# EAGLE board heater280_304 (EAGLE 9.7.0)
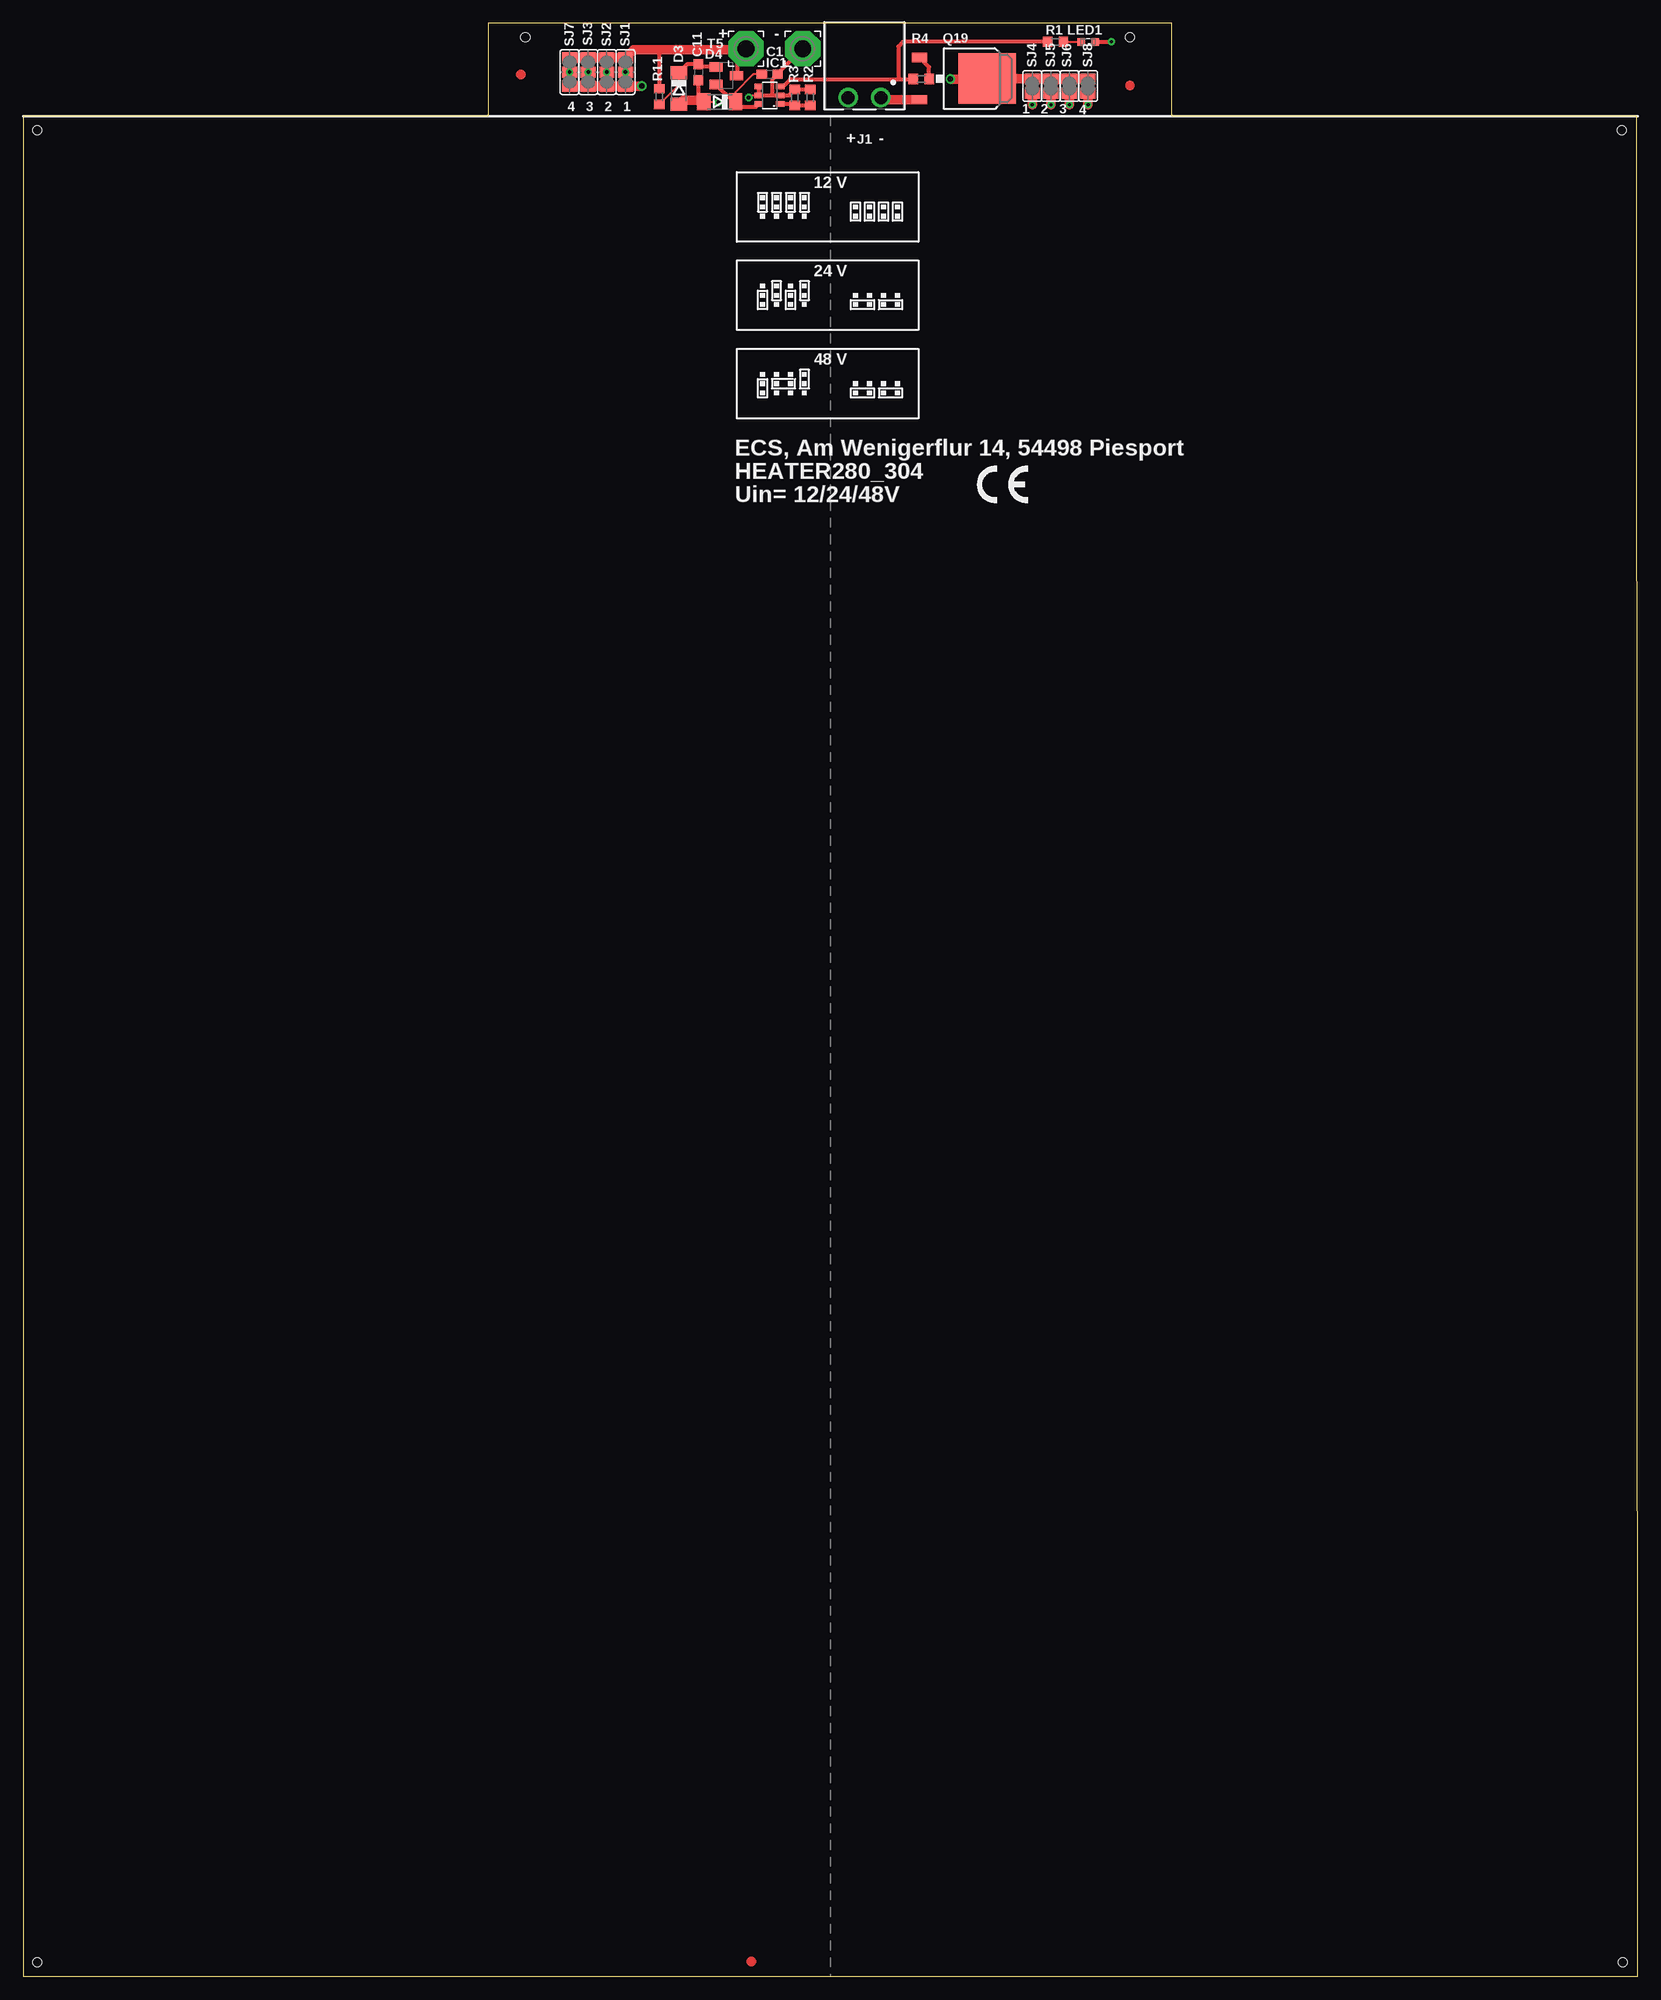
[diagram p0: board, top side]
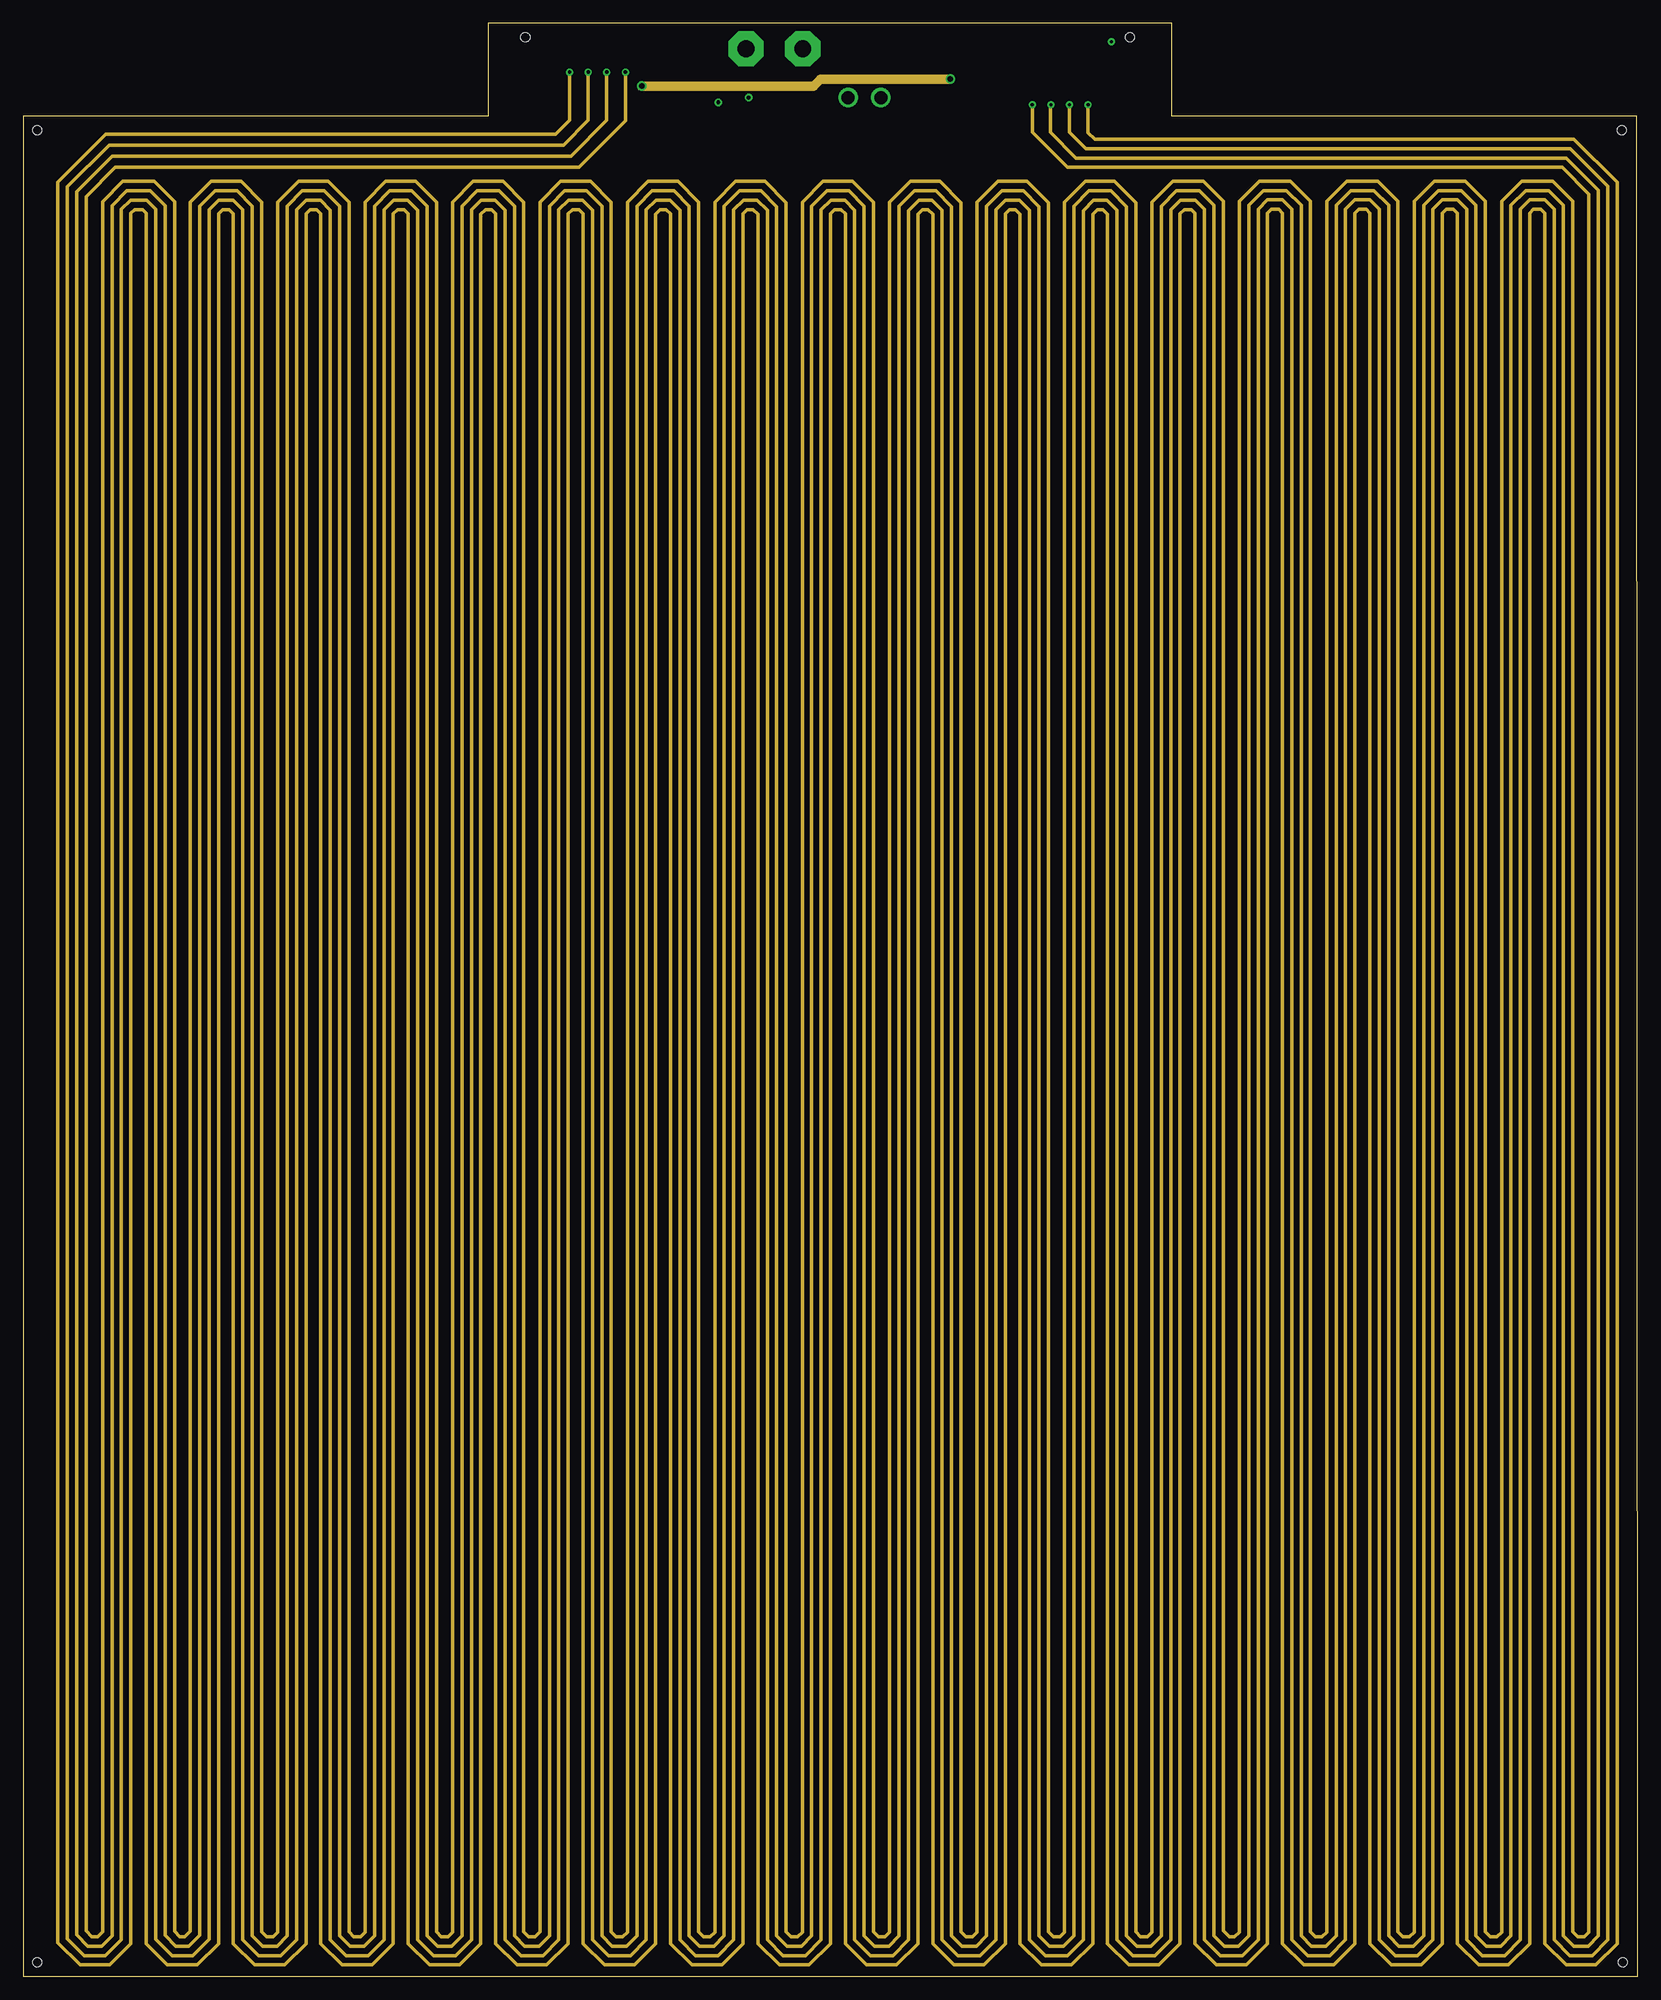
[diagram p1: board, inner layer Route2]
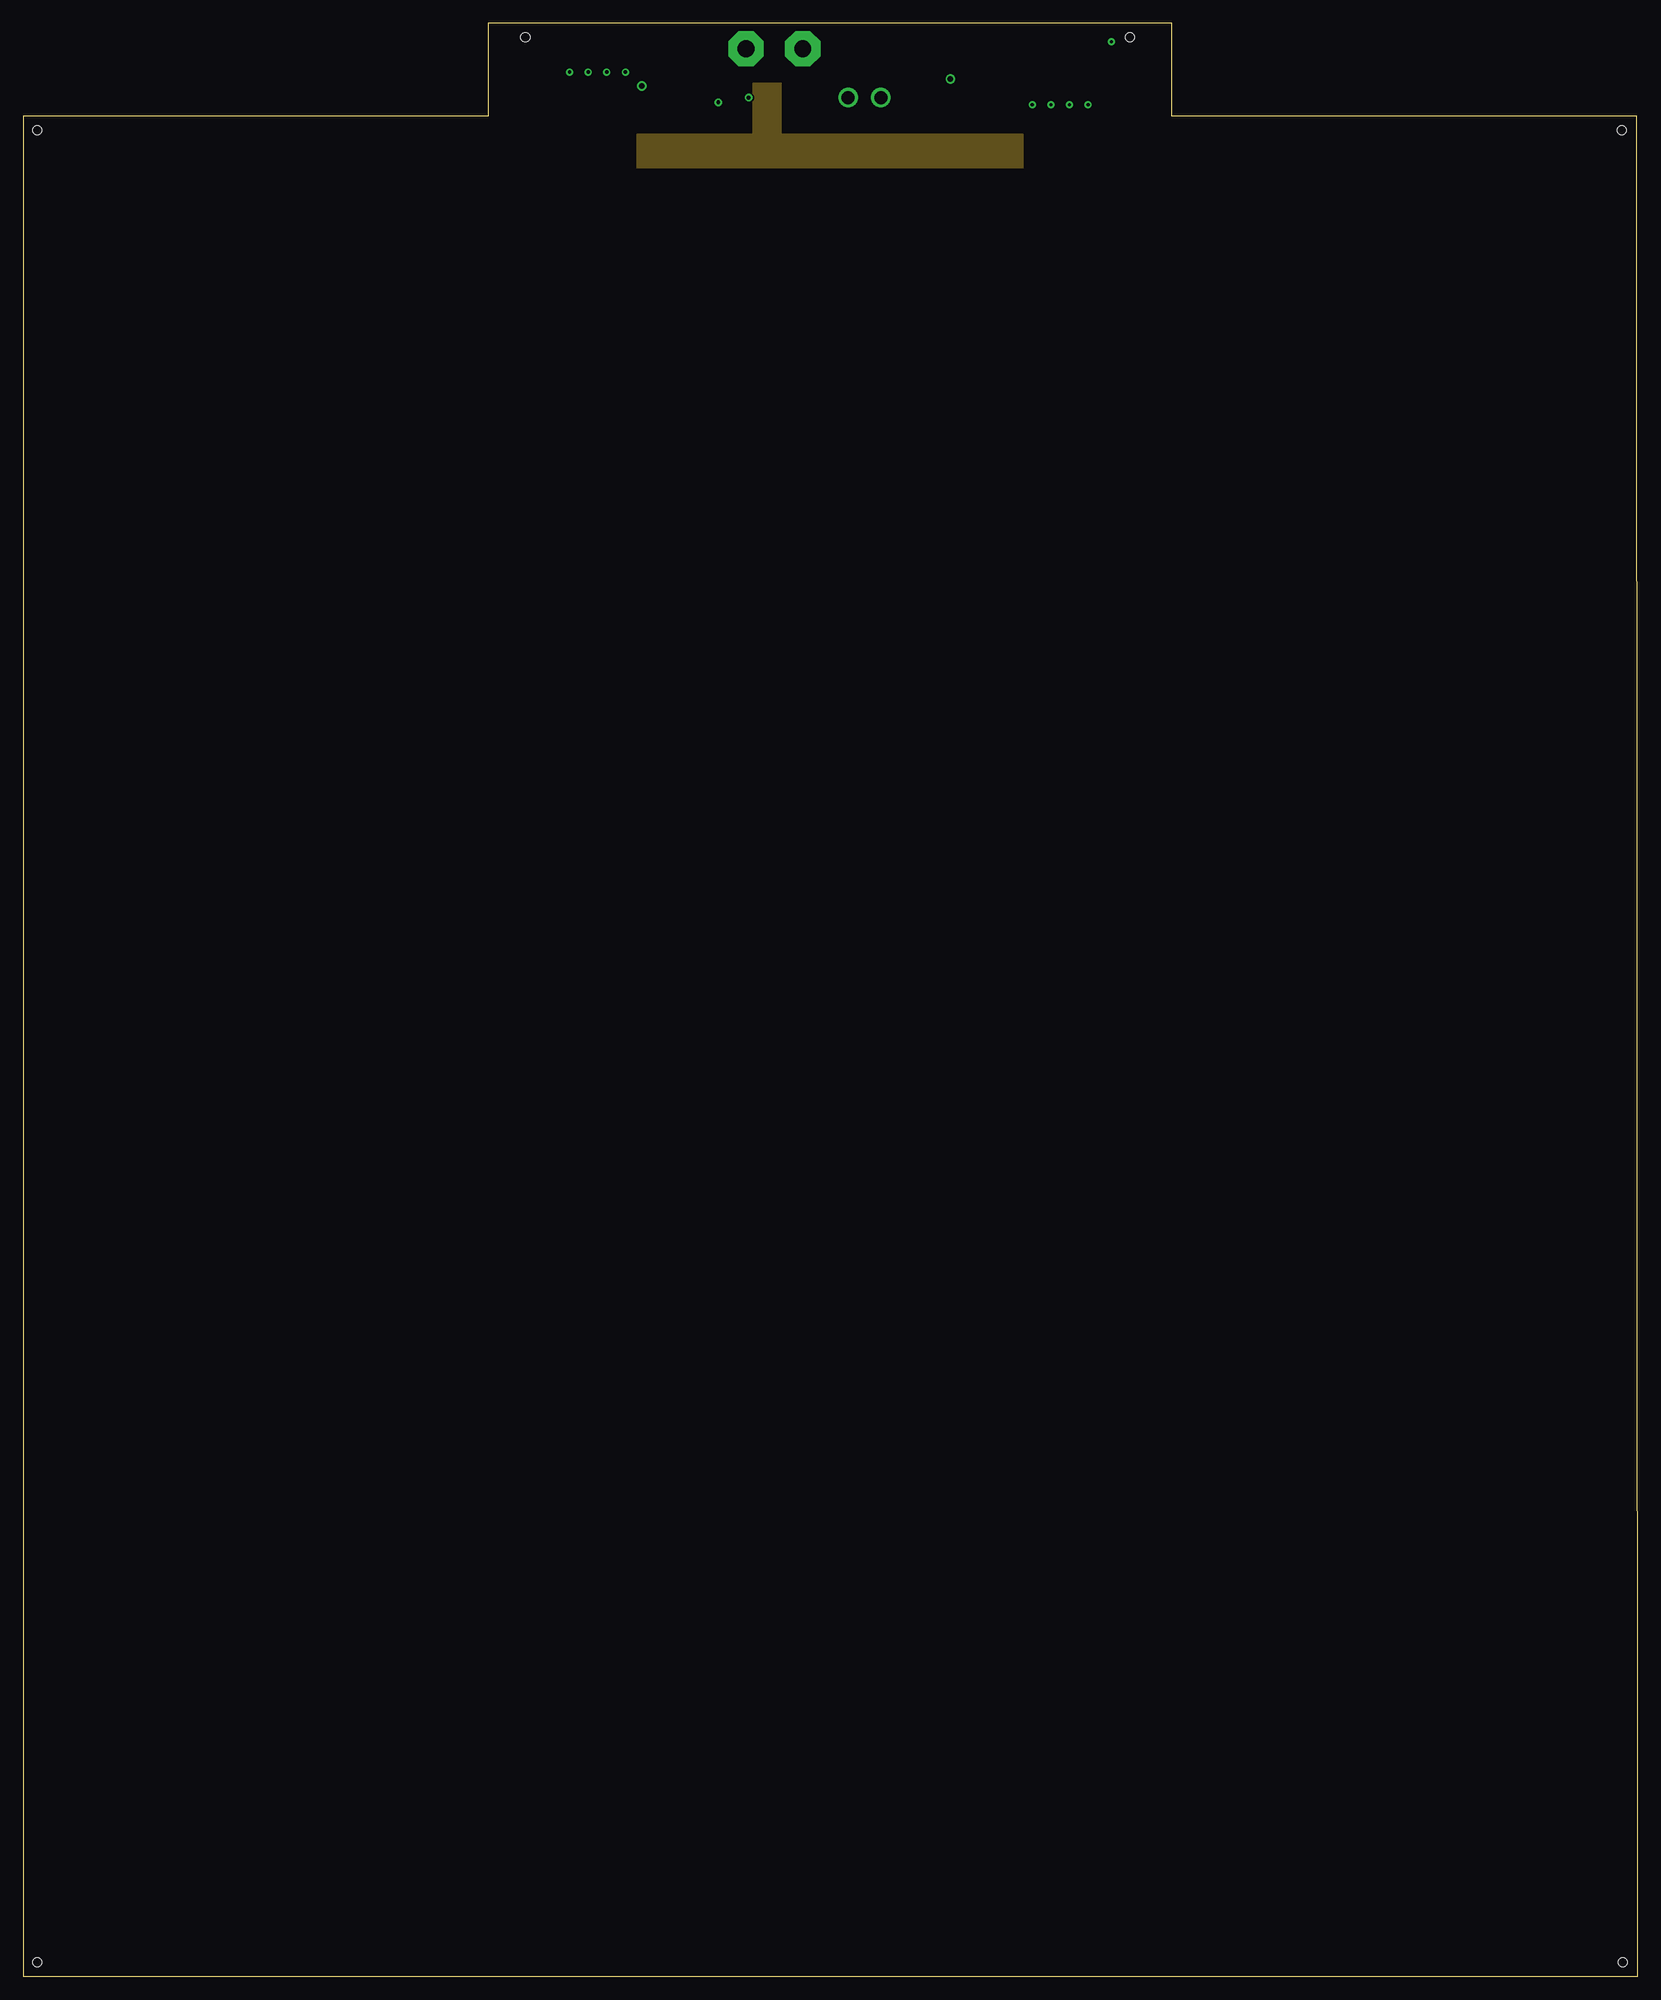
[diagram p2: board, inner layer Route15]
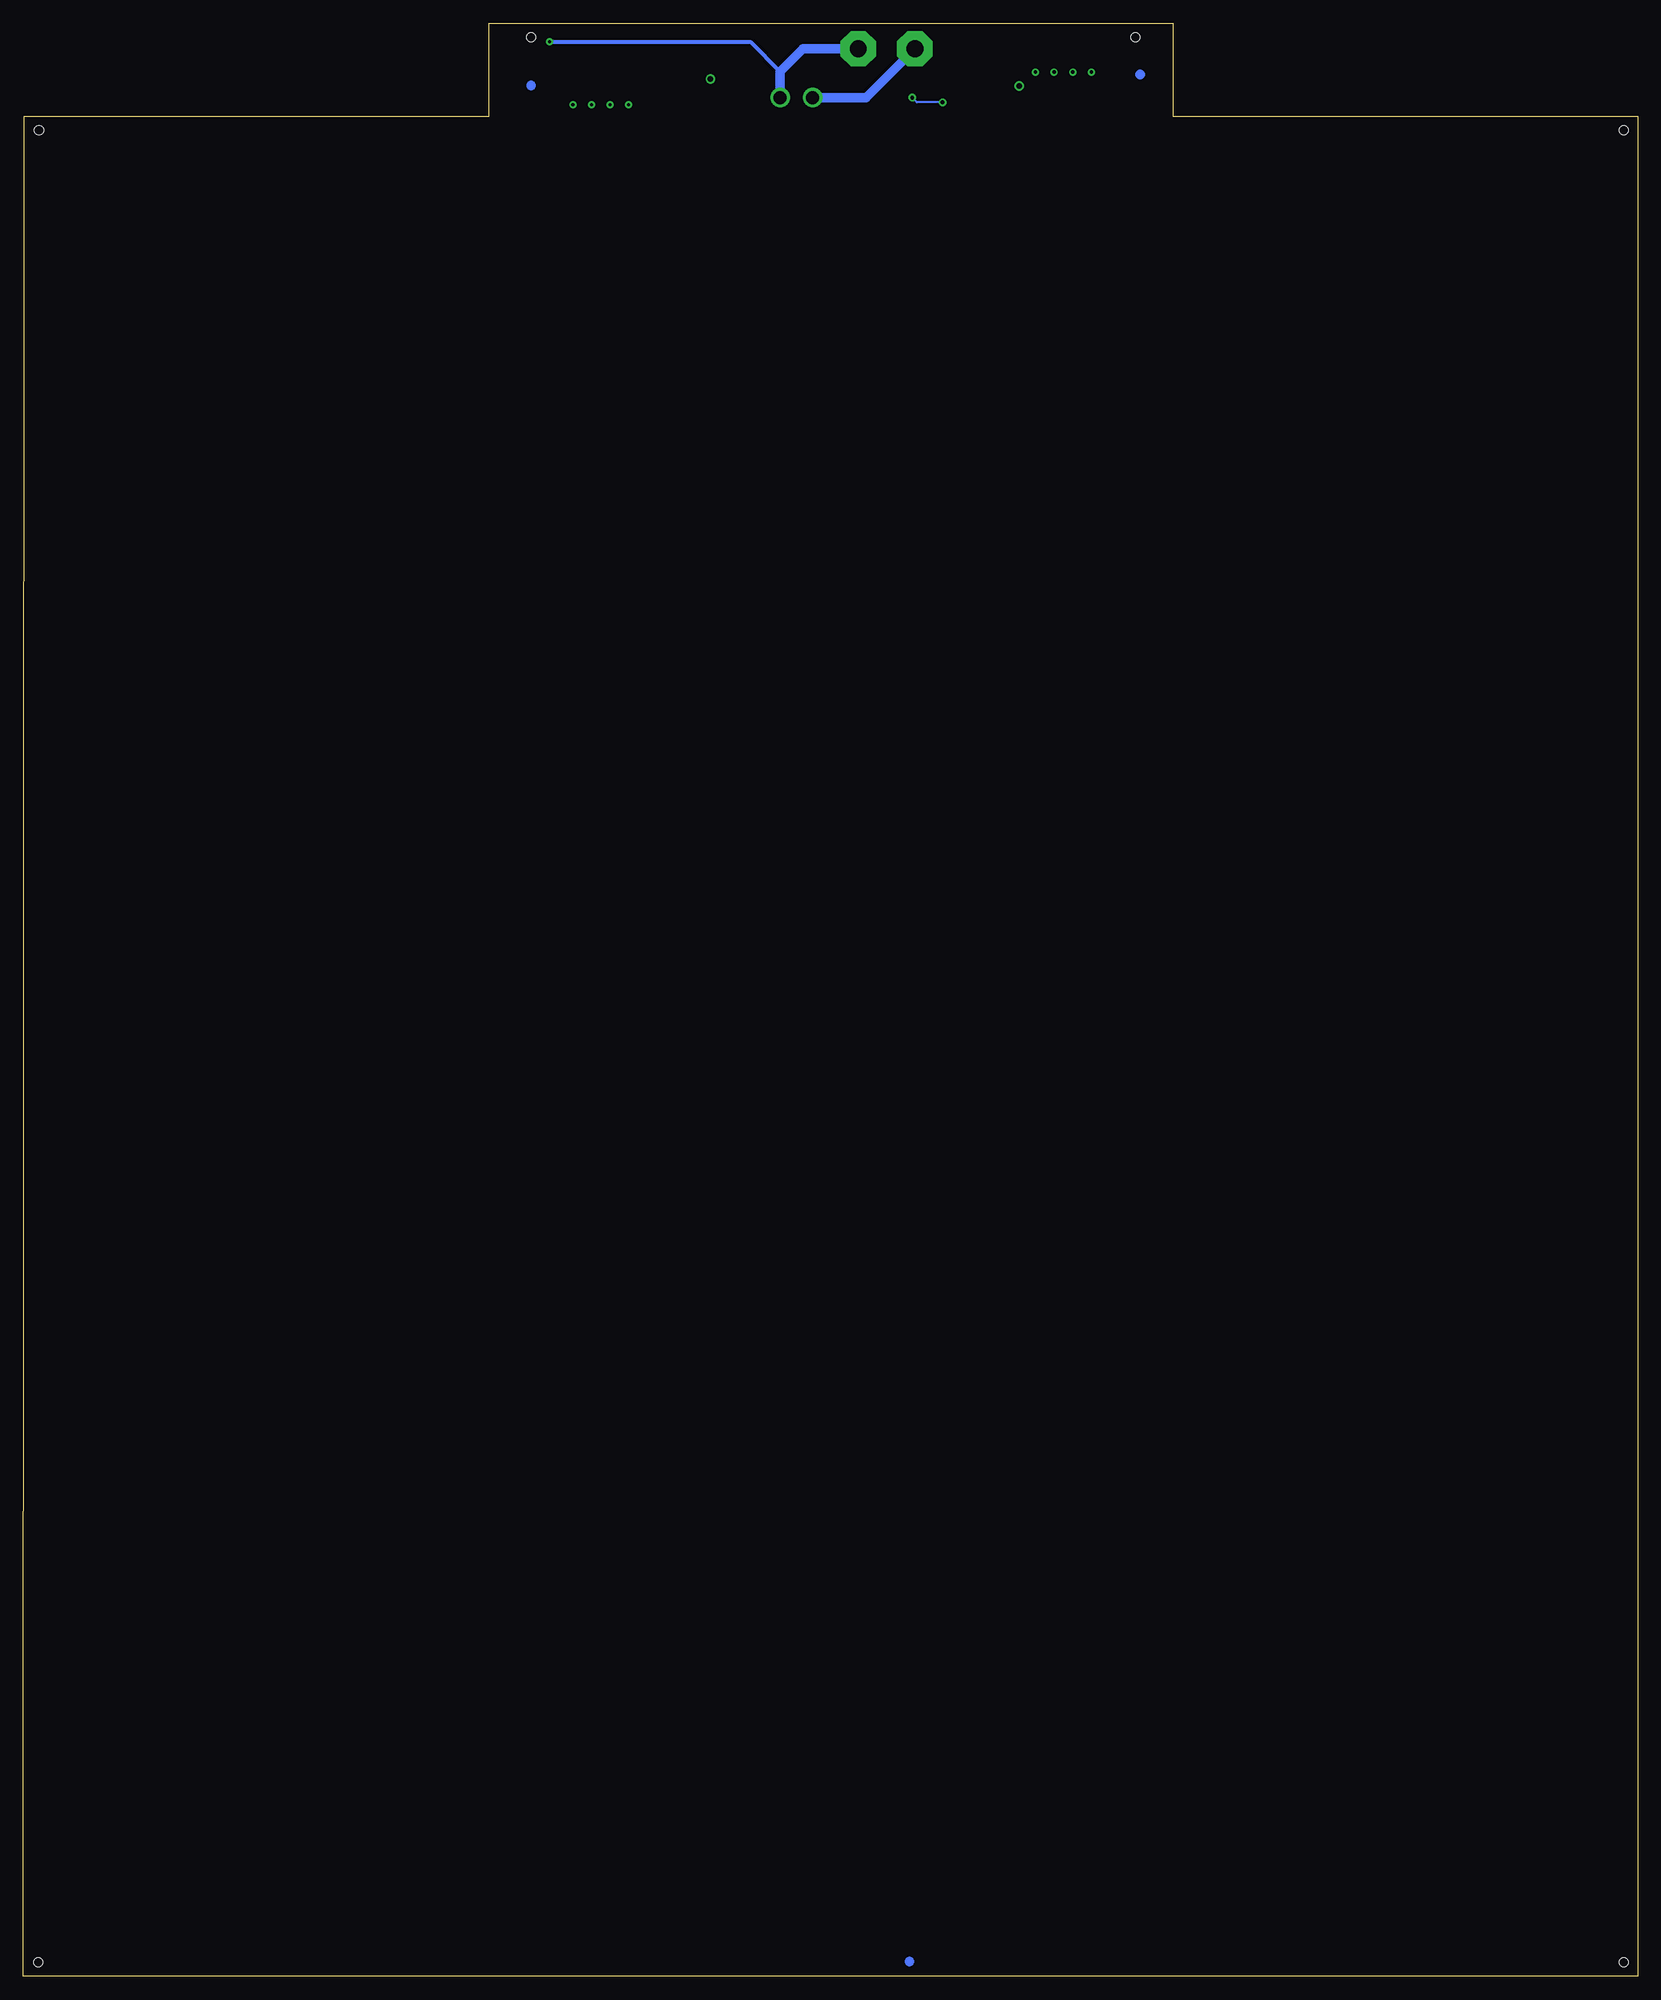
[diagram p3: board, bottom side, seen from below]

Size 173.6 x 210 mm. Coordinates in mm from the lower left corner, seen from the top.
Outline: 0,0 173.6,0 173.5,200 123.5,200 123.5,210 50,210 50,200 0,200 0,0
Copper layers (1+2*15+16): Top 0.035mm / dielectric 1.5mm / Route2 0.0175mm / dielectric 0.15mm / Route15 0.0175mm / dielectric 0.2mm / Bottom 0.035mm
Design rules "Fusion Electronics Design Rules": minimum track width 6mil, minimum drill 0.35mm, track to track 6mil, track to pad 6mil, pad to pad 6mil, via to via 6mil, smd to smd 6mil, copper to edge 40mil, drill to drill 6mil, minimum pad ring 10mil, minimum via ring 8mil, stop-mask expansion 4mil, vias tented up to drill 0mil, thermal gap 10mil
Holes 1 mm at 1.5,198.5 54,208.5 119,208.5 171.9,198.5 1.5,1.5 172,1.5

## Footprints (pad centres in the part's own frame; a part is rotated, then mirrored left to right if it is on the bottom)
C0603 = smd 1.1 x 1: 1 -0.85,0; 2 0.85,0
SOD80C = smd 1.4 x 1.8: A 1.7,0; C -1.7,0
SOT23-6 = smd 0.6 x 0.9: 1 -0.95,-1.15; 2 0,-1.15; 3 0.95,-1.15; 4 0.95,1.15; 5 0,1.15; 6 -0.95,1.15
691322110002 = drill 1.4: 1 -1.75,0; 2 1.75,0
SML0603 = smd 0.8 x 0.8: A 0.75,0; C -0.75,0
3,81/1,4 = drill 1.8 pad 3.81 octagon: 1 0,0
D-PACK = smd 1 x 1.6: 1 -2.28,-4.8; 3 2.28,-4.8 | smd 5.4 x 6.2: 4 0,2.5
R0603 = smd 1 x 1.1: 1 -0.85,0; 2 0.85,0
SJ_2 = smd 1.168 x 1.6: 1 -1.524,0; 2 0,0; 3 1.524,0
SJ = smd 1.168 x 1.6: 1 -0.762,0; 2 0.762,0
SOT23-BEC = smd 1 x 1.4: B -0.95,-1.1; C 0,1.1; E 0.95,-1.1

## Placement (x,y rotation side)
C1  100n  [C0603]  80.27,204.52 0 top
C11  100n  [C0603]  72.6,204.73 270 top
D3  5V6  [SOD80C]  70.5,203 270 top
D4  5V1  [SOD80C]  74.88,201.55 180 top
IC1  MCP9510H  [SOT23-6]  80.25,202.25 90 top
J1  [691322110002]  90.46,202.01 180 top
LED1  [SML0603]  114.5,208 180 top
PAD1  [3,81/1,4]  77.72,207.26 0 top
PAD2  [3,81/1,4]  83.82,207.26 0 top
Q19  IRLR3110Z  [D-PACK]  101.16,204.05 270 top
R1  10k  [R0603]  111,208 180 top
R2  82k  [R0603]  84.64,202.02 270 top
R3  2M2  [R0603]  82.97,202.02 270 top
R4  1k  [R0603]  96.57,204 180 top
R11  100k  [R0603]  68.4,202.12 90 top
SJ1  [SJ_2]  64.75,204.75 90 top
SJ2  [SJ_2]  62.75,204.75 90 top
SJ3  [SJ_2]  60.75,204.75 90 top
SJ4  [SJ]  108.5,203.25 270 top
SJ5  [SJ]  110.5,203.25 270 top
SJ6  [SJ]  112.5,203.25 270 top
SJ7  [SJ_2]  58.75,204.75 90 top
SJ8  [SJ]  114.5,203.25 270 top
T5  BSR19A  [SOT23-BEC]  75.61,204.36 270 top
U$1  [CE-4MM]  102.5,158.38 0 top
U$2  [CIRCLE-1MM-3R]  53.5,204.5 0 top
U$3  [CIRCLE-1MM-3R]  119,203.3 0 top
U$4  [CIRCLE-1MM-3R]  78.3,1.6 0 top

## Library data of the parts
C1 C11 = rcl; PARTNO: C067; SPICEPREFIX: C
D3 = diode; PARTNO: D013
D4 = diode; PARTNO: D012
IC1 = mcp9509; PARTNO: IC333
J1 = Wurth_Connectors_WR-TBL Pluggable Connector; DATASHEET-URL: https://www.we-online.com/catalog/datasheet/691322110002.pdf; IR-UL: 10A; IR-VDE: 10.5A; MOUNT: THT; PART-NUMBER: 691322110002; PARTNO: CON212; PINS: 2; PITCH: 3.5mm; TYPE: Horizontal; WORKING-VOLTAGE-UL: 300V (AC); WORKING-VOLTAGE-VDE: 300V (AC)
LED1 = led; PARTNO: D078
PAD1 PAD2 = wirepad
Q19 = IRFR2607; PARTNO: T086
R1 R4 = rcl; PARTNO: R221; SPICEPREFIX: R
R2 = rcl; PARTNO: R243; SPICEPREFIX: R
R3 = rcl; PARTNO: R277; SPICEPREFIX: R
R11 = rcl; PARTNO: R245; SPICEPREFIX: R
SJ1-SJ8 = jumper
T5 = transistor-neu-to92; PARTNO: T056
U$1 = logo
U$2-U$4 = fidu

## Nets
+UB: J1.2 PAD1.1 R11.2 SJ1.3 SJ2.3 SJ3.3 SJ7.3 T5.C
GND: C1.2 C11.2 D3.A D4.A IC1.2 IC1.4 IC1.5 J1.1 LED1.C PAD2.1 Q19.3 R2.1 R3.1
N$1: IC1.3 R1.2 R4.2
N$2: SJ1.2 SJ4.2
N$3: C11.1 D3.C R11.1 T5.B
N$4: IC1.1 R2.2 R3.2
N$5: C1.1 D4.C IC1.6 T5.E
N$6: LED1.A R1.1
N$7: SJ2.2 SJ5.2
N$8: SJ3.2 SJ6.2
N$9: SJ7.2 SJ8.2
N$11: Q19.4 SJ1.1 SJ2.1 SJ3.1 SJ4.1 SJ5.1 SJ6.1 SJ7.1 SJ8.1
N$12: Q19.1 R4.1

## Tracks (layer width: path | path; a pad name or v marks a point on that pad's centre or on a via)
+UB
  Top 0.406: T5.C 76.75,204.4 76.75,206.29 77.61,207.15 PAD1.1 | R11.2 68.4,207.04 68.5,207.15
  Top 1.016: SJ7.3 SJ3.3 SJ2.3 SJ1.3 65.62,207.15 68.5,207.15 77.61,207.15
  Bottom 1.016: PAD1.1 82.97,202.01 J1.2
GND  (via drill 0.35, 0.4)
  Top 0.2: D4.A 74.7,201.55 v74.75,201.5 | v78,202 78.25,202.25 IC1.5
  Top 0.406: D4.A 72.6,202.13 C11.2 | 80.56,202.25 IC1.2 82.35,202.25 R3.1 R2.1 | 80.56,202.25 80.56,203.96 C1.2 81.12,204.56 PAD2.1 | IC1.4 IC1.5 80.56,202.25 | LED1.C v117,208
  Top 1.016: D3.A 70.95,201.75 72.98,201.75 D4.A | Q19.3 92.45,201.77 J1.1
  Bottom 0.2: v74.75,201.5 77.5,201.5 v78,202
  Bottom 0.406: v117,208 95.42,208 92.21,204.79
  Bottom 1.016: J1.1 92.21,204.79 89.74,207.26 PAD2.1
N$1
  Top 0.406: IC1.3 81.7,203.2 82.5,204 94.1,204 | 94.1,204 R4.2 | R1.2 94.6,208 94.1,207.5 94.1,204
N$2  (via drill 0.35, 0.35 pad 0.21)
  Top 1.016: SJ4.2 v108.5,201.25
  Route2 0.4: SJ1.2 64.75,199.52 59.79,194.5 9.9,194.5 6.75,191.35 6.75,4.87 7.37,4.26 8.01,4.26 8.54,4.78 8.54,190.82 10.71,192.99 14.09,192.99 16.26,190.82 16.26,4.82 16.84,4.25 17.38,4.25 17.97,4.84 17.97,190.76 20.2,192.99 23.41,192.99 25.63,190.77 25.63,4.77 26.16,4.25 26.86,4.25 27.37,4.75 27.37,190.76 29.6,192.99 32.79,192.99 35.03,190.75 35.03,4.77 35.55,4.25 36.26,4.25 36.77,4.75 36.77,190.77 38.99,192.99 42.19,192.99 44.43,190.75 44.43,4.77 44.95,4.25 45.66,4.25 46.17,4.75 46.17,190.76 48.4,192.99 51.59,192.99 53.83,190.75 53.83,4.77 54.35,4.25 55.05,4.25 55.35,4.55 55.57,4.77 55.57,190.76 57.8,192.99 60.99,192.99 63.23,190.75 63.23,4.77 63.75,4.25 64.47,4.25 64.97,4.75 64.97,190.76 67.2,192.99 70.39,192.99 72.63,190.75 72.63,4.77 73.16,4.25 73.86,4.25 74.37,4.75 74.37,190.76 76.6,192.99 79.75,192.99 82.03,190.72 82.03,4.77 82.56,4.25 83.26,4.25 83.77,4.75 83.77,190.76 86,192.99 89.19,192.99 91.43,190.75 91.43,4.77 91.95,4.25 92.66,4.25 93.17,4.75 93.17,190.76 95.4,192.99 98.56,192.99 100.83,190.72 100.83,4.77 101.35,4.25 102.07,4.25 102.57,4.75 102.57,190.76 104.8,192.99 107.95,192.99 110.23,190.72 110.23,4.77 110.75,4.25 111.46,4.25 111.97,4.75 111.97,190.76 114.2,192.99 117.36,192.99 119.63,190.72 119.63,4.77 120.16,4.25 120.86,4.25 121.37,4.75 121.37,190.76 123.6,192.99 126.89,192.99 129.03,190.85 129.03,4.92 129.7,4.25 130.26,4.25 130.77,4.75 130.77,190.85 132.94,193.03 136.25,193.03 138.43,190.85 138.43,4.77 138.96,4.25 139.66,4.25 140.17,4.75 140.17,190.85 142.34,193.03 145.66,193.03 147.83,190.85 147.83,4.77 148.35,4.25 149.06,4.25 149.57,4.75 149.57,190.85 151.75,193.03 155.06,193.03 157.23,190.85 157.23,4.77 157.75,4.25 158.46,4.25 158.97,4.75 158.97,190.85 161.15,193.03 164.46,193.03 166.63,190.85 166.63,4.77 167.16,4.25 167.86,4.25 168.37,4.75 168.37,191.63 165.5,194.5 112.3,194.5 108.5,198.3 v108.5,201.25
  other vias: 64.75,204.75
N$3
  Top 0.2: R11.1 70.5,203.37 D3.C
  Top 0.406: D3.C 71.38,205.58 C11.1 72.87,205.31 T5.B
N$4
  Top 0.406: IC1.1 82.97,201.3 R3.2 R2.2
N$5
  Top 0.2: C1.1 79.4,204.5 78.5,204.5 76.58,202.58 D4.C
  Top 0.406: T5.E 76.37,201.55 D4.C 76.83,201.3 76.95,201.3 77.25,201 78.77,201 IC1.6
N$6
  Top 0.2: R1.1 LED1.A
N$7  (via drill 0.35, 0.35 pad 0.21)
  Top 1.016: SJ5.2 v110.5,201.25
  Route2 0.4: SJ2.2 62.75,199.55 58.9,195.7 9.56,195.7 5.74,191.89 5.74,4.45 6.95,3.25 8.43,3.25 9.54,4.36 9.54,190.4 11.13,191.98 13.67,191.98 15.26,190.4 15.26,4.4 16.42,3.23 17.8,3.23 18.98,4.42 18.98,190.34 20.62,191.98 22.99,191.98 24.62,190.35 24.62,4.35 25.74,3.23 27.28,3.23 28.38,4.34 28.38,190.34 30.02,191.98 32.38,191.98 34.02,190.34 34.02,4.35 35.14,3.24 36.68,3.24 37.78,4.34 37.78,190.35 39.41,191.98 41.77,191.98 43.42,190.34 43.42,4.35 44.54,3.23 46.08,3.23 47.18,4.34 47.18,190.34 48.82,191.98 51.17,191.98 52.82,190.34 52.82,4.35 53.93,3.23 55.47,3.23 56.12,3.88 56.58,4.35 56.58,190.34 58.22,191.98 60.57,191.98 62.22,190.34 62.22,4.35 63.34,3.23 64.88,3.23 65.98,4.34 65.98,190.34 67.62,191.98 69.97,191.98 71.62,190.34 71.62,4.35 72.74,3.23 74.28,3.23 75.38,4.34 75.38,190.34 77.02,191.98 79.34,191.98 81.02,190.3 81.02,4.35 82.14,3.23 83.68,3.23 84.78,4.34 84.78,190.34 86.42,191.98 88.77,191.98 90.42,190.34 90.42,4.35 91.54,3.23 93.08,3.23 94.18,4.34 94.18,190.34 95.82,191.98 98.14,191.98 99.82,190.3 99.82,4.35 100.94,3.23 102.48,3.23 103.58,4.34 103.58,190.34 105.22,191.98 107.54,191.98 109.22,190.3 109.22,4.35 110.34,3.23 111.88,3.23 112.98,4.34 112.98,190.34 114.62,191.98 116.94,191.98 118.62,190.3 118.62,4.35 119.74,3.23 121.28,3.23 122.38,4.34 122.38,190.34 124.02,191.98 126.47,191.98 128.02,190.44 128.02,4.35 129.14,3.23 130.68,3.23 131.78,4.34 131.78,190.44 133.36,192.02 135.84,192.02 137.42,190.44 137.42,4.35 138.54,3.23 140.08,3.23 141.18,4.34 141.18,190.44 142.76,192.02 145.24,192.02 146.82,190.44 146.82,4.35 147.94,3.23 149.48,3.23 150.58,4.34 150.58,190.44 152.16,192.02 154.64,192.02 156.22,190.44 156.22,4.35 157.34,3.23 158.88,3.23 159.98,4.34 159.98,190.44 161.56,192.02 164.04,192.02 165.62,190.44 165.62,4.35 166.74,3.23 168.28,3.23 169.38,4.34 169.38,192.05 165.92,195.51 113.22,195.51 110.46,198.26 110.46,201.21 v110.5,201.25
  other vias: 62.75,204.75
N$8  (via drill 0.35, 0.35 pad 0.21)
  Top 1.016: SJ6.2 v112.5,201.25
  Route2 0.4: SJ3.2 60.75,199.55 58.1,196.9 9.23,196.9 4.74,192.41 4.74,4.03 6.54,2.23 8.84,2.23 10.55,3.94 10.55,189.98 11.54,190.97 13.26,190.97 14.24,189.98 14.24,3.98 16,2.23 18.22,2.23 19.99,4 19.99,189.93 21.04,190.97 22.57,190.97 23.61,189.94 23.61,3.93 25.32,2.23 27.7,2.23 29.39,3.92 29.39,189.93 30.43,190.97 31.96,190.97 33.01,189.92 33.01,3.93 34.72,2.23 37.1,2.23 38.79,3.92 38.79,189.94 39.83,190.97 41.36,190.97 42.41,189.92 42.41,3.93 44.12,2.23 46.5,2.23 48.19,3.92 48.19,189.93 49.24,190.97 50.76,190.97 51.81,189.92 51.81,3.93 53.52,2.23 55.88,2.23 57.59,3.93 57.59,189.93 58.64,190.97 60.16,190.97 61.21,189.92 61.21,3.93 62.92,2.23 65.3,2.23 66.99,3.92 66.99,189.93 68.04,190.97 69.56,190.97 70.61,189.92 70.61,3.93 72.32,2.23 74.7,2.23 76.39,3.92 76.39,189.93 77.44,190.97 78.92,190.97 80.01,189.88 80.01,3.93 81.72,2.23 84.1,2.23 85.79,3.92 85.79,189.93 86.84,190.97 88.36,190.97 89.41,189.92 89.41,3.93 91.12,2.23 93.5,2.23 95.19,3.92 95.19,189.86 96.3,190.97 97.72,190.97 98.81,189.88 98.81,3.93 100.52,2.23 102.9,2.23 104.59,3.92 104.59,189.93 105.64,190.97 107.12,190.97 108.21,189.88 108.21,3.93 109.92,2.23 112.3,2.23 113.99,3.92 113.99,189.86 115.1,190.97 116.52,190.97 117.61,189.88 117.61,3.93 119.32,2.23 121.7,2.23 123.39,3.92 123.39,189.93 124.44,190.97 126.06,190.97 127.01,190.02 127.01,3.93 128.72,2.23 131.1,2.23 132.79,3.92 132.79,190.02 133.78,191.01 135.42,191.01 136.41,190.02 136.41,3.93 138.12,2.23 140.5,2.23 142.19,3.92 142.19,190.02 143.18,191.01 144.82,191.01 145.81,190.02 145.81,3.93 147.52,2.23 149.9,2.23 151.59,3.92 151.59,190.02 152.58,191.01 154.22,191.01 155.21,190.02 155.21,3.93 156.92,2.23 159.3,2.23 160.99,3.92 160.99,190.02 161.98,191.01 163.62,191.01 164.61,190.02 164.61,3.93 166.32,2.23 168.7,2.23 170.39,3.92 170.39,192.47 166.34,196.52 114.28,196.52 112.5,198.3 v112.5,201.25
  other vias: 60.75,204.75
N$9  (via drill 0.35, 0.35 pad 0.21)
  Top 1.016: SJ8.2 v114.5,201.25
  Route2 0.4: SJ7.2 58.75,199.55 57.25,198.05 8.85,198.05 3.73,192.93 3.73,3.62 6.12,1.22 9.29,1.22 11.56,3.49 11.56,189.56 11.96,189.96 12.84,189.96 13.24,189.56 13.24,3.48 15.5,1.22 18.72,1.22 21,3.5 21,189.51 21.45,189.95 22.16,189.95 22.6,189.52 22.6,3.52 24.9,1.22 28.12,1.22 30.4,3.5 30.4,189.51 30.85,189.95 31.55,189.95 32,189.5 32,3.52 34.3,1.22 37.52,1.22 39.8,3.5 39.8,189.52 40.24,189.96 40.94,189.96 41.4,189.5 41.4,3.52 43.7,1.22 46.92,1.22 49.2,3.5 49.2,189.46 49.7,189.96 50.34,189.96 50.8,189.5 50.8,3.5 53.1,1.22 56.3,1.22 58.6,3.5 58.6,189.51 59.05,189.95 59.75,189.95 60.2,189.5 60.2,3.52 62.5,1.22 65.72,1.22 68,3.5 68,189.46 68.5,189.96 69.14,189.96 69.6,189.5 69.6,3.52 71.9,1.22 75.12,1.22 77.4,3.5 77.4,189.51 77.86,189.96 78.5,189.96 79,189.46 79,3.52 81.3,1.22 84.52,1.22 86.8,3.5 86.8,189.51 87.25,189.96 87.94,189.96 88.4,189.5 88.4,3.52 90.7,1.22 93.92,1.22 96.2,3.5 96.2,189.44 96.72,189.96 97.3,189.96 97.8,189.46 97.8,3.52 100.1,1.22 103.32,1.22 105.6,3.5 105.6,189.51 106.06,189.96 106.7,189.96 107.2,189.46 107.2,3.52 109.5,1.22 112.72,1.22 115,3.5 115,189.44 115.52,189.96 116.1,189.96 116.6,189.46 116.6,3.52 118.9,1.22 122.12,1.22 124.4,3.5 124.4,189.51 124.86,189.96 125.64,189.96 126,189.6 126,3.52 128.3,1.22 131.52,1.22 133.8,3.5 133.8,189.6 134.2,190 135,190 135.4,189.6 135.4,3.52 137.7,1.22 140.92,1.22 143.2,3.5 143.2,189.6 143.6,190 144.4,190 144.8,189.6 144.8,3.52 147.1,1.22 150.32,1.22 152.6,3.5 152.6,189.6 153,190 153.8,190 154.2,189.6 154.2,3.52 156.5,1.22 159.72,1.22 162,3.5 162,189.6 162.4,190 163.2,190 163.6,189.6 163.6,3.52 165.9,1.22 169.12,1.22 171.4,3.5 171.4,192.88 166.75,197.53 115.22,197.53 114.5,198.25 v114.5,201.25
  other vias: 58.75,204.75
N$10
  pour Route15: 78.48,198.04 78.46,198.02 78.42,198 66,198 66,194.5 107.5,194.5 107.5,198 81.58,198 81.54,198.02 81.52,198.04 81.5,198.08 81.5,203.5 78.5,203.5 78.5,198.08
N$11  (via drill 0.6)
  Top 1.016: SJ7.1 SJ3.1 SJ2.1 SJ1.1 66.48,203.23 v66.5,203.25 | SJ8.1 SJ6.1 SJ5.1 SJ4.1 104.65,204.01 103.66,205 Q19.4 103.61,204 v99.7,204
  Route2 1.016: v66.5,203.25 85,203.25 85.75,204 v99.7,204
N$12
  Top 0.406: R4.1 97.42,205.27 Q19.1

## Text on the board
tPlace: + | - | 4 | 3 | 2 | 1 | 1 | 2 | 3 | 4 | + | - | 12 V | 24 V | 48 V | ECS, Am Wenigerflur 14, 54498 Piesport | HEATER280_304 | Uin= 12/24/48V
